FUNCTION FC 90 : VOID
TITLE =GESTIONE ALLARMI / AVVISI
AUTHOR : MassimoZ
VERSION : 0.1

BEGIN
NETWORK
TITLE ======== Avvisi Generali =======



NETWORK
TITLE =Avviso: Manca Marcia Generale
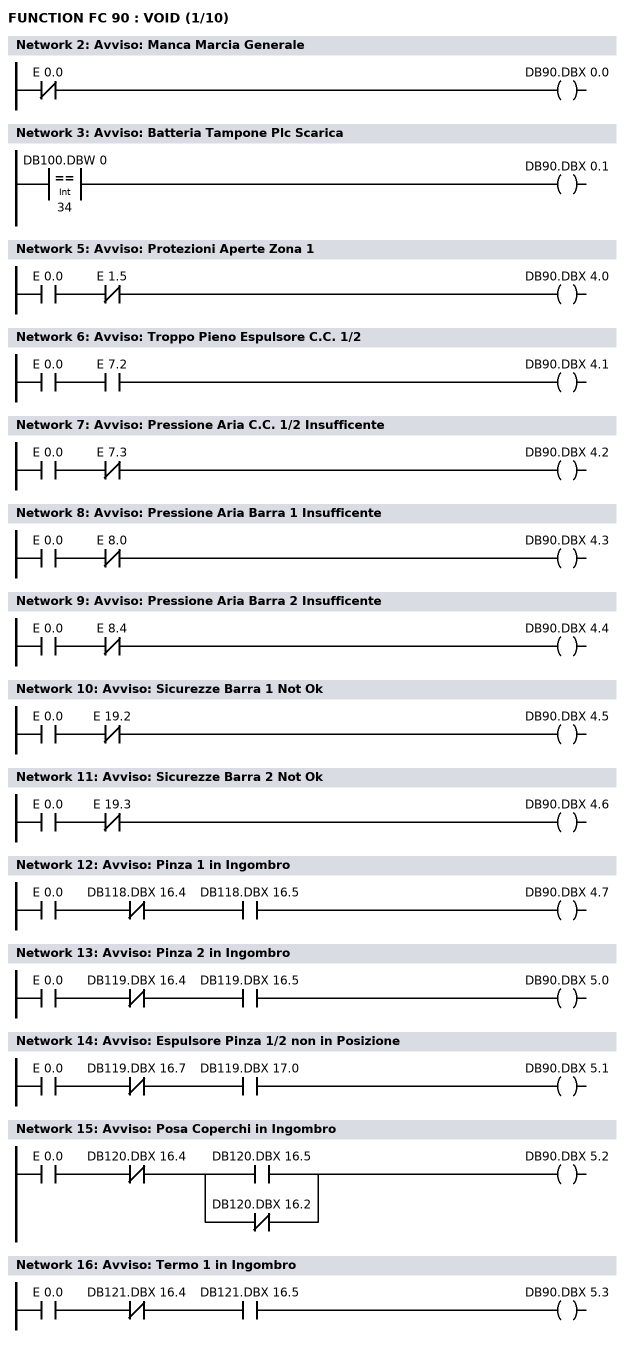
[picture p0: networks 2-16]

      UN    E      0.0;
      =     DB90.DBX    0.0;
NETWORK
TITLE =Avviso: Batteria Tampone Plc Scarica

      L     DB100.DBW    0;
      L     34;
      ==I   ;
      =     DB90.DBX    0.1;
NETWORK
TITLE ======== Avvisi Zona 1 =======



NETWORK
TITLE =Avviso: Protezioni Aperte Zona 1

      U     E      0.0;
      UN    E      1.5;
      =     DB90.DBX    4.0;
NETWORK
TITLE =Avviso: Troppo Pieno Espulsore C.C. 1/2

      U     E      0.0;
      U     E      7.2;
      =     DB90.DBX    4.1;
NETWORK
TITLE =Avviso: Pressione Aria C.C. 1/2 Insufficente

      U     E      0.0;
      UN    E      7.3;
      =     DB90.DBX    4.2;
NETWORK
TITLE =Avviso: Pressione Aria Barra 1 Insufficente

      U     E      0.0;
      UN    E      8.0;
      =     DB90.DBX    4.3;
NETWORK
TITLE =Avviso: Pressione Aria Barra 2 Insufficente

      U     E      0.0;
      UN    E      8.4;
      =     DB90.DBX    4.4;
NETWORK
TITLE =Avviso: Sicurezze Barra 1 Not Ok

      U     E      0.0;
      UN    E     19.2;
      =     DB90.DBX    4.5;
NETWORK
TITLE =Avviso: Sicurezze Barra 2 Not Ok

      U     E      0.0;
      UN    E     19.3;
      =     DB90.DBX    4.6;
NETWORK
TITLE =Avviso: Pinza 1 in Ingombro

      U     E      0.0;
      UN    DB118.DBX   16.4;
      U     DB118.DBX   16.5;
      =     DB90.DBX    4.7;
NETWORK
TITLE =Avviso: Pinza 2 in Ingombro

      U     E      0.0;
      UN    DB119.DBX   16.4;
      U     DB119.DBX   16.5;
      =     DB90.DBX    5.0;
NETWORK
TITLE =Avviso: Espulsore Pinza 1/2 non in Posizione

      U     E      0.0;
      UN    DB119.DBX   16.7;
      U     DB119.DBX   17.0;
      =     DB90.DBX    5.1;
NETWORK
TITLE =Avviso: Posa Coperchi in Ingombro

      U     E      0.0;
      UN    DB120.DBX   16.4;
      U(    ;
      O     DB120.DBX   16.5;
      ON    DB120.DBX   16.2;
      )     ;
      =     DB90.DBX    5.2;
NETWORK
TITLE =Avviso: Termo 1 in Ingombro

      U     E      0.0;
      UN    DB121.DBX   16.4;
      U     DB121.DBX   16.5;
      =     DB90.DBX    5.3;
NETWORK
TITLE =Avviso: Termo 2 in Ingombro
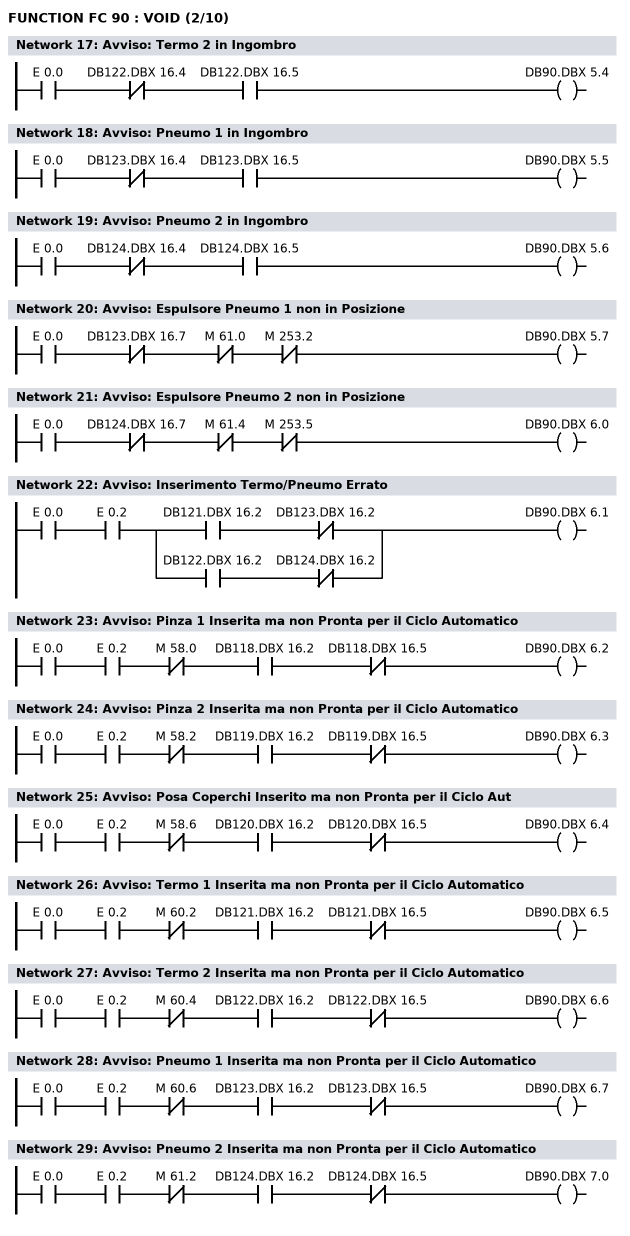
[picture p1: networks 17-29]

      U     E      0.0;
      UN    DB122.DBX   16.4;
      U     DB122.DBX   16.5;
      =     DB90.DBX    5.4;
NETWORK
TITLE =Avviso: Pneumo 1 in Ingombro

      U     E      0.0;
      UN    DB123.DBX   16.4;
      U     DB123.DBX   16.5;
      =     DB90.DBX    5.5;
NETWORK
TITLE =Avviso: Pneumo 2 in Ingombro

      U     E      0.0;
      UN    DB124.DBX   16.4;
      U     DB124.DBX   16.5;
      =     DB90.DBX    5.6;
NETWORK
TITLE =Avviso: Espulsore Pneumo 1 non in Posizione

      U     E      0.0;
      UN    DB123.DBX   16.7;
      UN    M     61.0;
      UN    M    253.2;
      =     DB90.DBX    5.7;
NETWORK
TITLE =Avviso: Espulsore Pneumo 2 non in Posizione

      U     E      0.0;
      UN    DB124.DBX   16.7;
      UN    M     61.4;
      UN    M    253.5;
      =     DB90.DBX    6.0;
NETWORK
TITLE =Avviso: Inserimento Termo/Pneumo Errato

      U     E      0.0;
      U     E      0.2;
      U(    ;
      U     DB121.DBX   16.2;
      UN    DB123.DBX   16.2;
      O     ;
      U     DB122.DBX   16.2;
      UN    DB124.DBX   16.2;
      )     ;
      =     DB90.DBX    6.1;
NETWORK
TITLE =Avviso: Pinza 1 Inserita ma non Pronta per il Ciclo Automatico

      U     E      0.0;
      U     E      0.2;
      UN    M     58.0;
      U     DB118.DBX   16.2;
      UN    DB118.DBX   16.5;
      =     DB90.DBX    6.2;
NETWORK
TITLE =Avviso: Pinza 2 Inserita ma non Pronta per il Ciclo Automatico

      U     E      0.0;
      U     E      0.2;
      UN    M     58.2;
      U     DB119.DBX   16.2;
      UN    DB119.DBX   16.5;
      =     DB90.DBX    6.3;
NETWORK
TITLE =Avviso: Posa Coperchi Inserito ma non Pronta per il Ciclo Aut

      U     E      0.0;
      U     E      0.2;
      UN    M     58.6;
      U     DB120.DBX   16.2;
      UN    DB120.DBX   16.5;
      =     DB90.DBX    6.4;
NETWORK
TITLE =Avviso: Termo 1 Inserita ma non Pronta per il Ciclo Automatico

      U     E      0.0;
      U     E      0.2;
      UN    M     60.2;
      U     DB121.DBX   16.2;
      UN    DB121.DBX   16.5;
      =     DB90.DBX    6.5;
NETWORK
TITLE =Avviso: Termo 2 Inserita ma non Pronta per il Ciclo Automatico

      U     E      0.0;
      U     E      0.2;
      UN    M     60.4;
      U     DB122.DBX   16.2;
      UN    DB122.DBX   16.5;
      =     DB90.DBX    6.6;
NETWORK
TITLE =Avviso: Pneumo 1 Inserita ma non Pronta per il Ciclo Automatico

      U     E      0.0;
      U     E      0.2;
      UN    M     60.6;
      U     DB123.DBX   16.2;
      UN    DB123.DBX   16.5;
      =     DB90.DBX    6.7;
NETWORK
TITLE =Avviso: Pneumo 2 Inserita ma non Pronta per il Ciclo Automatico

      U     E      0.0;
      U     E      0.2;
      UN    M     61.2;
      U     DB124.DBX   16.2;
      UN    DB124.DBX   16.5;
      =     DB90.DBX    7.0;
NETWORK
TITLE =Avviso: Zona Pulsantiera 1 non Pronta per il Ciclo Automatico
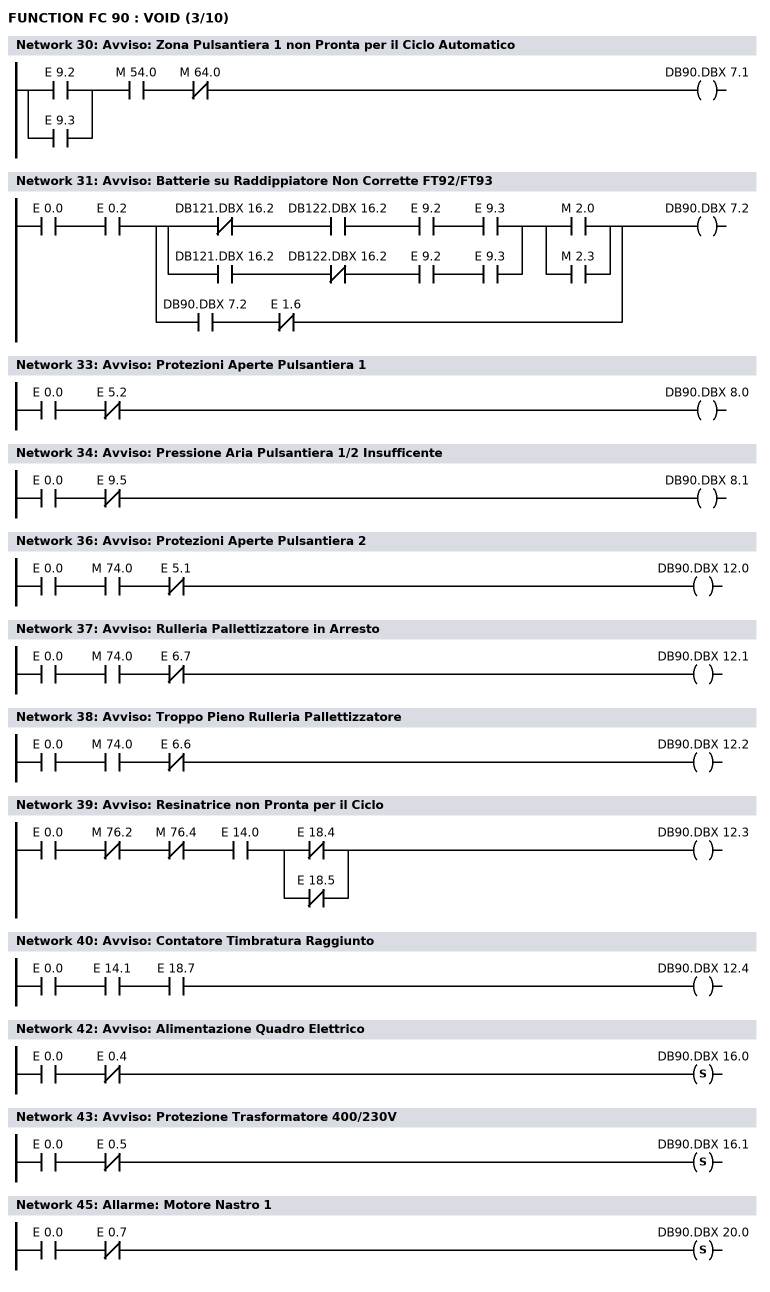
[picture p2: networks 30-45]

      U(    ;
      O     E      9.2;
      O     E      9.3;
      )     ;
      U     M     54.0;
      UN    M     64.0;
      =     DB90.DBX    7.1;
NETWORK
TITLE =Avviso: Batterie su Raddippiatore Non Corrette FT92/FT93

      U     E      0.0;
      U     E      0.2;
      U(    ;
      U(    ;
      UN    DB121.DBX   16.2;
      U     DB122.DBX   16.2;
      U     E      9.2;
      U     E      9.3;
      O     ;
      U     DB121.DBX   16.2;
      UN    DB122.DBX   16.2;
      U     E      9.2;
      U     E      9.3;
      )     ;
      U(    ;
      O     M      2.0;
      O     M      2.3;
      )     ;
      O     ;
      U     DB90.DBX    7.2;
      UN    E      1.6;
      )     ;
      =     DB90.DBX    7.2;
NETWORK
TITLE ======== Avvisi Pulsantiera 1 =======



NETWORK
TITLE =Avviso: Protezioni Aperte Pulsantiera 1

      U     E      0.0;
      UN    E      5.2;
      =     DB90.DBX    8.0;
NETWORK
TITLE =Avviso: Pressione Aria Pulsantiera 1/2 Insufficente

      U     E      0.0;
      UN    E      9.5;
      =     DB90.DBX    8.1;
NETWORK
TITLE ======== Avvisi Pulsantiera 2 =======



NETWORK
TITLE =Avviso: Protezioni Aperte Pulsantiera 2

      U     E      0.0;
      U     M     74.0;
      UN    E      5.1;
      =     DB90.DBX   12.0;
NETWORK
TITLE =Avviso: Rulleria Pallettizzatore in Arresto

      U     E      0.0;
      U     M     74.0;
      UN    E      6.7;
      =     DB90.DBX   12.1;
NETWORK
TITLE =Avviso: Troppo Pieno Rulleria Pallettizzatore

      U     E      0.0;
      U     M     74.0;
      UN    E      6.6;
      =     DB90.DBX   12.2;
NETWORK
TITLE =Avviso: Resinatrice non Pronta per il Ciclo

      U     E      0.0;
      UN    M     76.2;
      UN    M     76.4;
      U     E     14.0;
      U(    ;
      ON    E     18.4;
      ON    E     18.5;
      )     ;
      =     DB90.DBX   12.3;
NETWORK
TITLE =Avviso: Contatore Timbratura Raggiunto

      U     E      0.0;
      U     E     14.1;
      U     E     18.7;
      =     DB90.DBX   12.4;
NETWORK
TITLE ======== Allarmi Generali =======



NETWORK
TITLE =Avviso: Alimentazione Quadro Elettrico

      U     E      0.0;
      UN    E      0.4;
      S     DB90.DBX   16.0;
NETWORK
TITLE =Avviso: Protezione Trasformatore 400/230V

      U     E      0.0;
      UN    E      0.5;
      S     DB90.DBX   16.1;
NETWORK
TITLE ======== Allarmi Zona 1 =======



NETWORK
TITLE =Allarme: Motore Nastro 1

      U     E      0.0;
      UN    E      0.7;
      S     DB90.DBX   20.0;
NETWORK
TITLE =Allarme: Motore Regolazione Altezza C.C.1
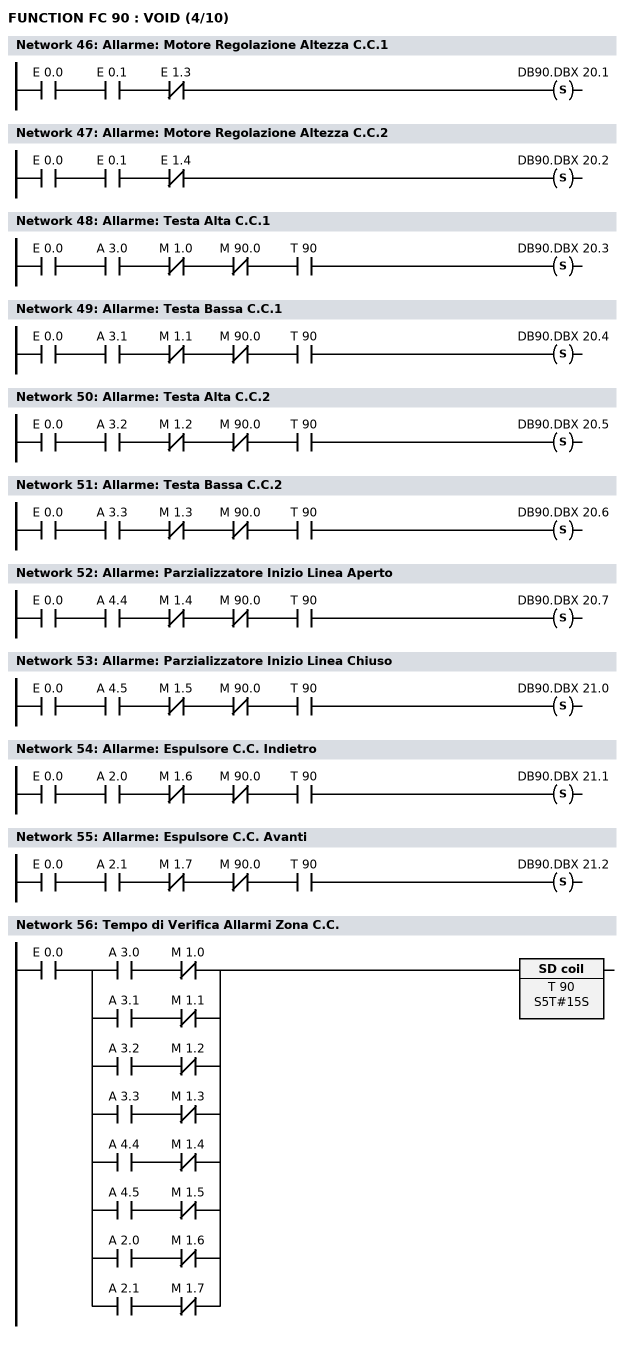
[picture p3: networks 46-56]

      U     E      0.0;
      U     E      0.1;
      UN    E      1.3;
      S     DB90.DBX   20.1;
NETWORK
TITLE =Allarme: Motore Regolazione Altezza C.C.2

      U     E      0.0;
      U     E      0.1;
      UN    E      1.4;
      S     DB90.DBX   20.2;
NETWORK
TITLE =Allarme: Testa Alta C.C.1

      U     E      0.0;
      U     A      3.0;
      UN    M      1.0;
      UN    M     90.0;
      U     T     90;
      S     DB90.DBX   20.3;
NETWORK
TITLE =Allarme: Testa Bassa C.C.1

      U     E      0.0;
      U     A      3.1;
      UN    M      1.1;
      UN    M     90.0;
      U     T     90;
      S     DB90.DBX   20.4;
NETWORK
TITLE =Allarme: Testa Alta C.C.2

      U     E      0.0;
      U     A      3.2;
      UN    M      1.2;
      UN    M     90.0;
      U     T     90;
      S     DB90.DBX   20.5;
NETWORK
TITLE =Allarme: Testa Bassa C.C.2

      U     E      0.0;
      U     A      3.3;
      UN    M      1.3;
      UN    M     90.0;
      U     T     90;
      S     DB90.DBX   20.6;
NETWORK
TITLE =Allarme: Parzializzatore Inizio Linea Aperto

      U     E      0.0;
      U     A      4.4;
      UN    M      1.4;
      UN    M     90.0;
      U     T     90;
      S     DB90.DBX   20.7;
NETWORK
TITLE =Allarme: Parzializzatore Inizio Linea Chiuso

      U     E      0.0;
      U     A      4.5;
      UN    M      1.5;
      UN    M     90.0;
      U     T     90;
      S     DB90.DBX   21.0;
NETWORK
TITLE =Allarme: Espulsore C.C. Indietro

      U     E      0.0;
      U     A      2.0;
      UN    M      1.6;
      UN    M     90.0;
      U     T     90;
      S     DB90.DBX   21.1;
NETWORK
TITLE =Allarme: Espulsore C.C. Avanti

      U     E      0.0;
      U     A      2.1;
      UN    M      1.7;
      UN    M     90.0;
      U     T     90;
      S     DB90.DBX   21.2;
NETWORK
TITLE =Tempo di Verifica Allarmi Zona C.C.

      U     E      0.0;
      U(    ;
      U     A      3.0;
      UN    M      1.0;
      O     ;
      U     A      3.1;
      UN    M      1.1;
      O     ;
      U     A      3.2;
      UN    M      1.2;
      O     ;
      U     A      3.3;
      UN    M      1.3;
      O     ;
      U     A      4.4;
      UN    M      1.4;
      O     ;
      U     A      4.5;
      UN    M      1.5;
      O     ;
      U     A      2.0;
      UN    M      1.6;
      O     ;
      U     A      2.1;
      UN    M      1.7;
      )     ;
      L     S5T#15S;
      SE    T     90;
NETWORK
TITLE =Presenza Allarme Barra 1/2
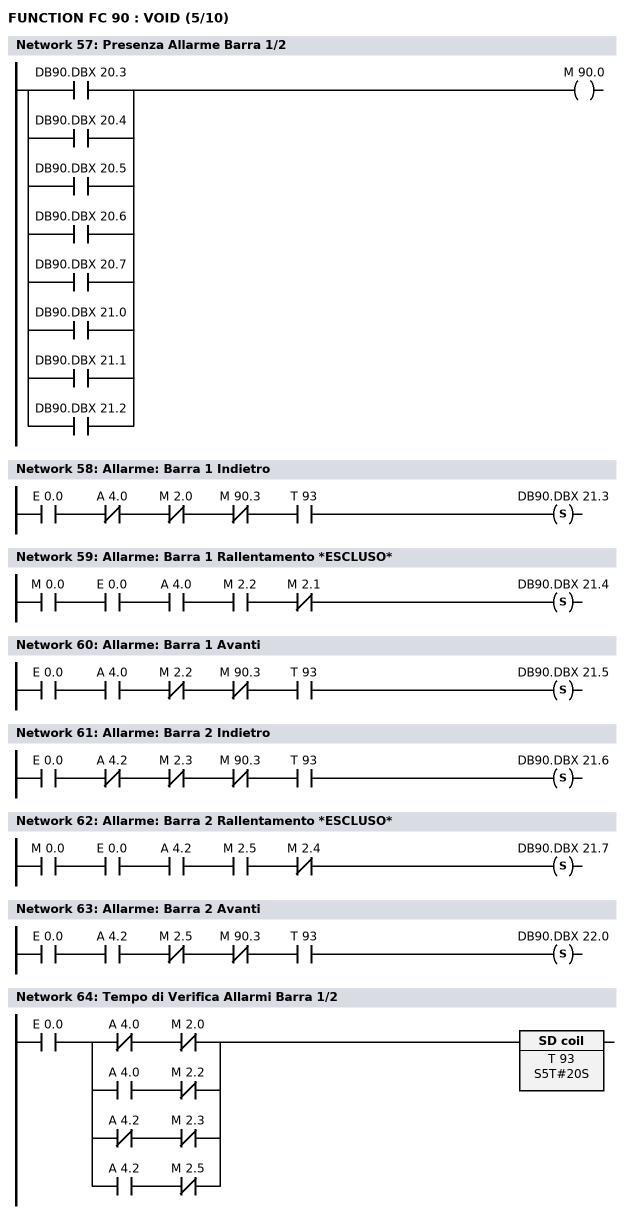
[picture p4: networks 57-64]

      O     DB90.DBX   20.3;
      O     DB90.DBX   20.4;
      O     DB90.DBX   20.5;
      O     DB90.DBX   20.6;
      O     DB90.DBX   20.7;
      O     DB90.DBX   21.0;
      O     DB90.DBX   21.1;
      O     DB90.DBX   21.2;
      =     M     90.0;
NETWORK
TITLE =Allarme: Barra 1 Indietro

      U     E      0.0;
      UN    A      4.0;
      UN    M      2.0;
      UN    M     90.3;
      U     T     93;
      S     DB90.DBX   21.3;
NETWORK
TITLE =Allarme: Barra 1 Rallentamento *ESCLUSO*

      U     M      0.0;
      U     E      0.0;
      U     A      4.0;
      U     M      2.2;
      UN    M      2.1;
      S     DB90.DBX   21.4;
NETWORK
TITLE =Allarme: Barra 1 Avanti

      U     E      0.0;
      U     A      4.0;
      UN    M      2.2;
      UN    M     90.3;
      U     T     93;
      S     DB90.DBX   21.5;
NETWORK
TITLE =Allarme: Barra 2 Indietro

      U     E      0.0;
      UN    A      4.2;
      UN    M      2.3;
      UN    M     90.3;
      U     T     93;
      S     DB90.DBX   21.6;
NETWORK
TITLE =Allarme: Barra 2 Rallentamento *ESCLUSO*

      U     M      0.0;
      U     E      0.0;
      U     A      4.2;
      U     M      2.5;
      UN    M      2.4;
      S     DB90.DBX   21.7;
NETWORK
TITLE =Allarme: Barra 2 Avanti

      U     E      0.0;
      U     A      4.2;
      UN    M      2.5;
      UN    M     90.3;
      U     T     93;
      S     DB90.DBX   22.0;
NETWORK
TITLE =Tempo di Verifica Allarmi Barra 1/2

      U     E      0.0;
      U(    ;
      UN    A      4.0;
      UN    M      2.0;
      O     ;
      U     A      4.0;
      UN    M      2.2;
      O     ;
      UN    A      4.2;
      UN    M      2.3;
      O     ;
      U     A      4.2;
      UN    M      2.5;
      )     ;
      L     S5T#20S;
      SE    T     93;
NETWORK
TITLE =Presenza Allarme Barra 1/2
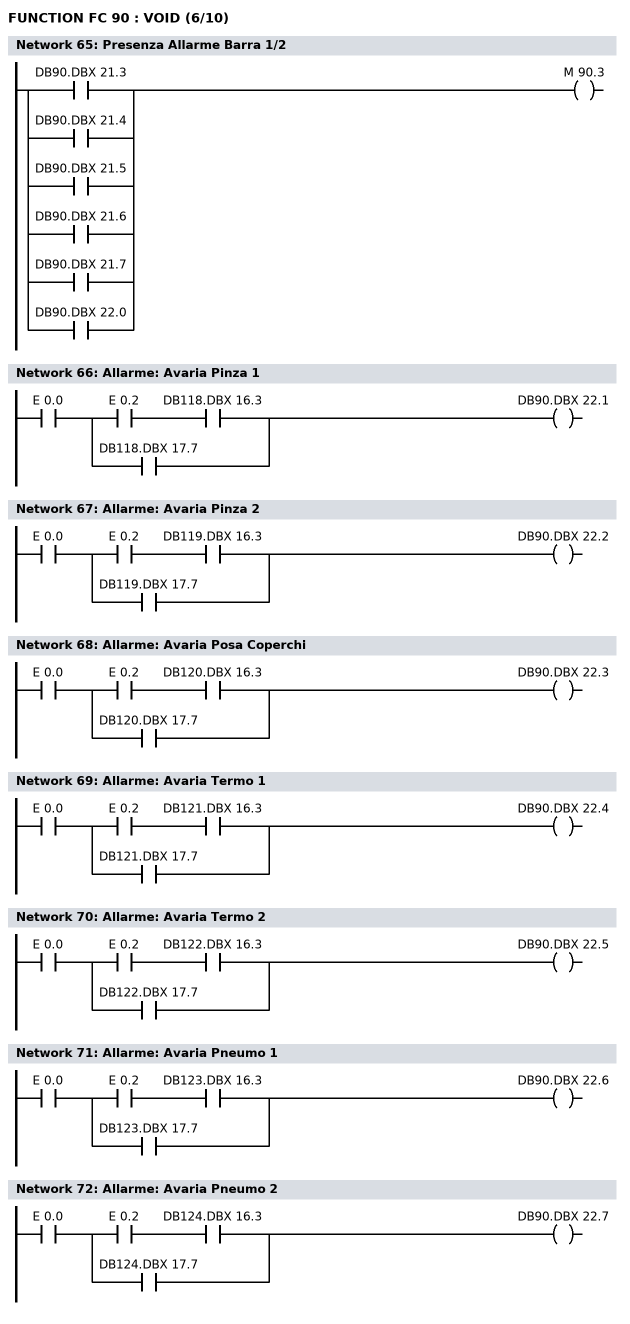
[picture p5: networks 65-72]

      O     DB90.DBX   21.3;
      O     DB90.DBX   21.4;
      O     DB90.DBX   21.5;
      O     DB90.DBX   21.6;
      O     DB90.DBX   21.7;
      O     DB90.DBX   22.0;
      =     M     90.3;
NETWORK
TITLE =Allarme: Avaria Pinza 1

      U     E      0.0;
      U(    ;
      U     E      0.2;
      U     DB118.DBX   16.3;
      O     DB118.DBX   17.7;
      )     ;
      =     DB90.DBX   22.1;
NETWORK
TITLE =Allarme: Avaria Pinza 2

      U     E      0.0;
      U(    ;
      U     E      0.2;
      U     DB119.DBX   16.3;
      O     DB119.DBX   17.7;
      )     ;
      =     DB90.DBX   22.2;
NETWORK
TITLE =Allarme: Avaria Posa Coperchi

      U     E      0.0;
      U(    ;
      U     E      0.2;
      U     DB120.DBX   16.3;
      O     DB120.DBX   17.7;
      )     ;
      =     DB90.DBX   22.3;
NETWORK
TITLE =Allarme: Avaria Termo 1

      U     E      0.0;
      U(    ;
      U     E      0.2;
      U     DB121.DBX   16.3;
      O     DB121.DBX   17.7;
      )     ;
      =     DB90.DBX   22.4;
NETWORK
TITLE =Allarme: Avaria Termo 2

      U     E      0.0;
      U(    ;
      U     E      0.2;
      U     DB122.DBX   16.3;
      O     DB122.DBX   17.7;
      )     ;
      =     DB90.DBX   22.5;
NETWORK
TITLE =Allarme: Avaria Pneumo 1

      U     E      0.0;
      U(    ;
      U     E      0.2;
      U     DB123.DBX   16.3;
      O     DB123.DBX   17.7;
      )     ;
      =     DB90.DBX   22.6;
NETWORK
TITLE =Allarme: Avaria Pneumo 2

      U     E      0.0;
      U(    ;
      U     E      0.2;
      U     DB124.DBX   16.3;
      O     DB124.DBX   17.7;
      )     ;
      =     DB90.DBX   22.7;
NETWORK
TITLE ======== Allarmi Pulsantiera 1 =======



NETWORK
TITLE =Allarme: Inverter
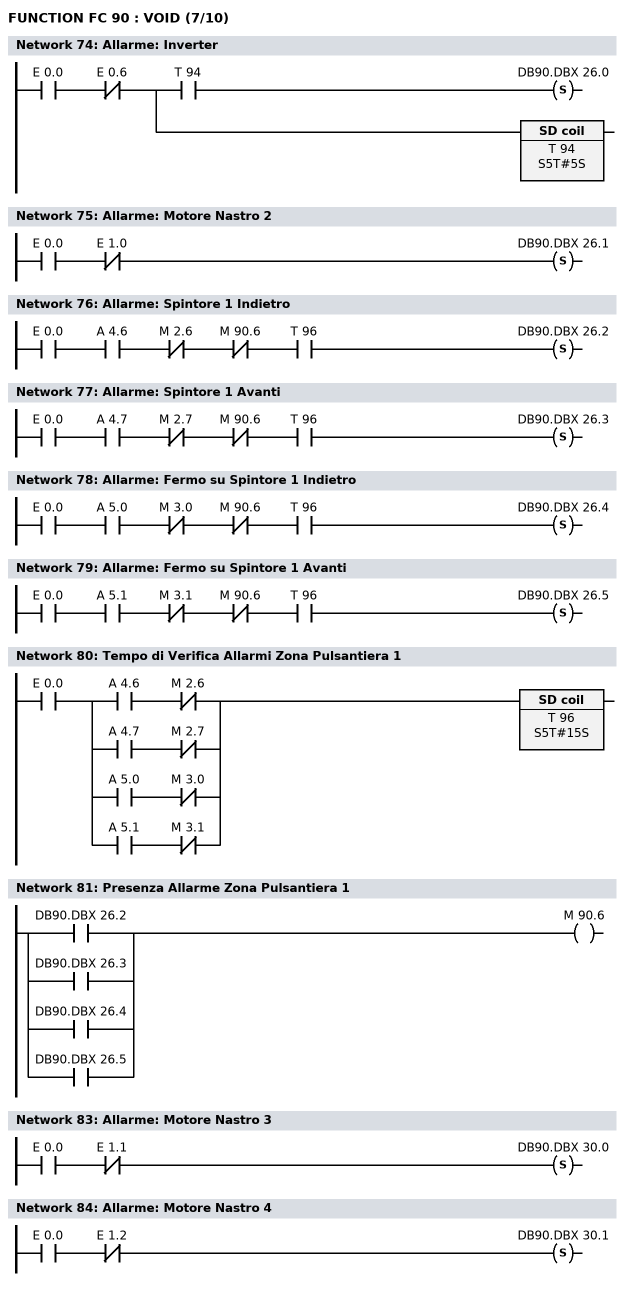
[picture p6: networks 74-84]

      U     E      0.0;
      UN    E      0.6;
      =     L      0.0;
      U     L      0.0;
      U     T     94;
      S     DB90.DBX   26.0;
      U     L      0.0;
      BLD   102;
      L     S5T#5S;
      SE    T     94;
NETWORK
TITLE =Allarme: Motore Nastro 2

      U     E      0.0;
      UN    E      1.0;
      S     DB90.DBX   26.1;
NETWORK
TITLE =Allarme: Spintore 1 Indietro

      U     E      0.0;
      U     A      4.6;
      UN    M      2.6;
      UN    M     90.6;
      U     T     96;
      S     DB90.DBX   26.2;
NETWORK
TITLE =Allarme: Spintore 1 Avanti

      U     E      0.0;
      U     A      4.7;
      UN    M      2.7;
      UN    M     90.6;
      U     T     96;
      S     DB90.DBX   26.3;
NETWORK
TITLE =Allarme: Fermo su Spintore 1 Indietro

      U     E      0.0;
      U     A      5.0;
      UN    M      3.0;
      UN    M     90.6;
      U     T     96;
      S     DB90.DBX   26.4;
NETWORK
TITLE =Allarme: Fermo su Spintore 1 Avanti

      U     E      0.0;
      U     A      5.1;
      UN    M      3.1;
      UN    M     90.6;
      U     T     96;
      S     DB90.DBX   26.5;
NETWORK
TITLE =Tempo di Verifica Allarmi Zona Pulsantiera 1

      U     E      0.0;
      U(    ;
      U     A      4.6;
      UN    M      2.6;
      O     ;
      U     A      4.7;
      UN    M      2.7;
      O     ;
      U     A      5.0;
      UN    M      3.0;
      O     ;
      U     A      5.1;
      UN    M      3.1;
      )     ;
      L     S5T#15S;
      SE    T     96;
NETWORK
TITLE =Presenza Allarme Zona Pulsantiera 1

      O     DB90.DBX   26.2;
      O     DB90.DBX   26.3;
      O     DB90.DBX   26.4;
      O     DB90.DBX   26.5;
      =     M     90.6;
NETWORK
TITLE ======== Allarmi Pulsantiera 2 =======



NETWORK
TITLE =Allarme: Motore Nastro 3

      U     E      0.0;
      UN    E      1.1;
      S     DB90.DBX   30.0;
NETWORK
TITLE =Allarme: Motore Nastro 4

      U     E      0.0;
      UN    E      1.2;
      S     DB90.DBX   30.1;
NETWORK
TITLE =Allarme: Parzializzatore SX Nastro 3 Aperto
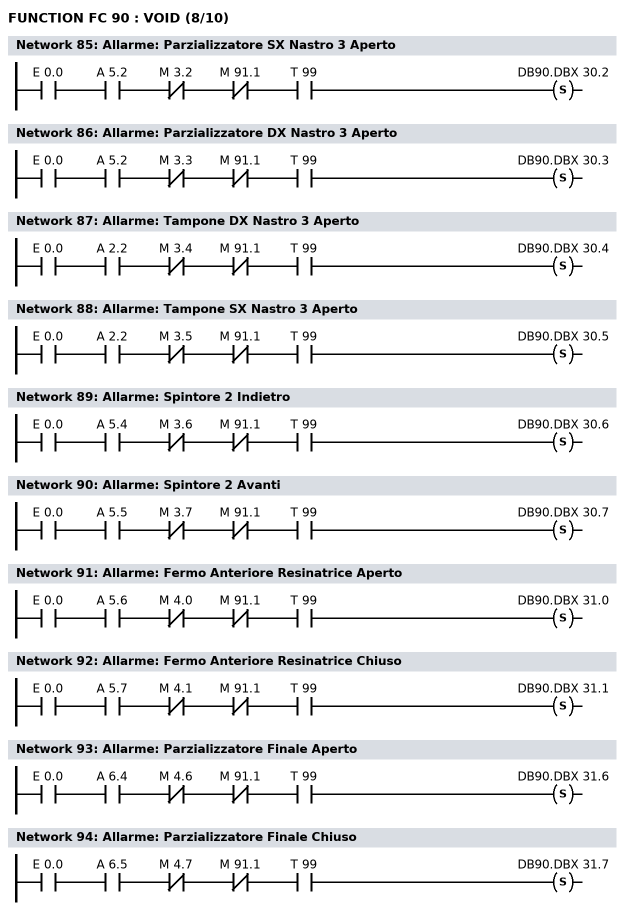
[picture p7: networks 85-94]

      U     E      0.0;
      U     A      5.2;
      UN    M      3.2;
      UN    M     91.1;
      U     T     99;
      S     DB90.DBX   30.2;
NETWORK
TITLE =Allarme: Parzializzatore DX Nastro 3 Aperto

      U     E      0.0;
      U     A      5.2;
      UN    M      3.3;
      UN    M     91.1;
      U     T     99;
      S     DB90.DBX   30.3;
NETWORK
TITLE =Allarme: Tampone DX Nastro 3 Aperto

      U     E      0.0;
      U     A      2.2;
      UN    M      3.4;
      UN    M     91.1;
      U     T     99;
      S     DB90.DBX   30.4;
NETWORK
TITLE =Allarme: Tampone SX Nastro 3 Aperto

      U     E      0.0;
      U     A      2.2;
      UN    M      3.5;
      UN    M     91.1;
      U     T     99;
      S     DB90.DBX   30.5;
NETWORK
TITLE =Allarme: Spintore 2 Indietro

      U     E      0.0;
      U     A      5.4;
      UN    M      3.6;
      UN    M     91.1;
      U     T     99;
      S     DB90.DBX   30.6;
NETWORK
TITLE =Allarme: Spintore 2 Avanti

      U     E      0.0;
      U     A      5.5;
      UN    M      3.7;
      UN    M     91.1;
      U     T     99;
      S     DB90.DBX   30.7;
NETWORK
TITLE =Allarme: Fermo Anteriore Resinatrice Aperto

      U     E      0.0;
      U     A      5.6;
      UN    M      4.0;
      UN    M     91.1;
      U     T     99;
      S     DB90.DBX   31.0;
NETWORK
TITLE =Allarme: Fermo Anteriore Resinatrice Chiuso

      U     E      0.0;
      U     A      5.7;
      UN    M      4.1;
      UN    M     91.1;
      U     T     99;
      S     DB90.DBX   31.1;
NETWORK
TITLE =Allarme: Parzializzatore Finale Aperto

      U     E      0.0;
      U     A      6.4;
      UN    M      4.6;
      UN    M     91.1;
      U     T     99;
      S     DB90.DBX   31.6;
NETWORK
TITLE =Allarme: Parzializzatore Finale Chiuso

      U     E      0.0;
      U     A      6.5;
      UN    M      4.7;
      UN    M     91.1;
      U     T     99;
      S     DB90.DBX   31.7;
NETWORK
TITLE =Tempo di Verifica Allarmi Parz/Fermi Zona Pulsantiera 2
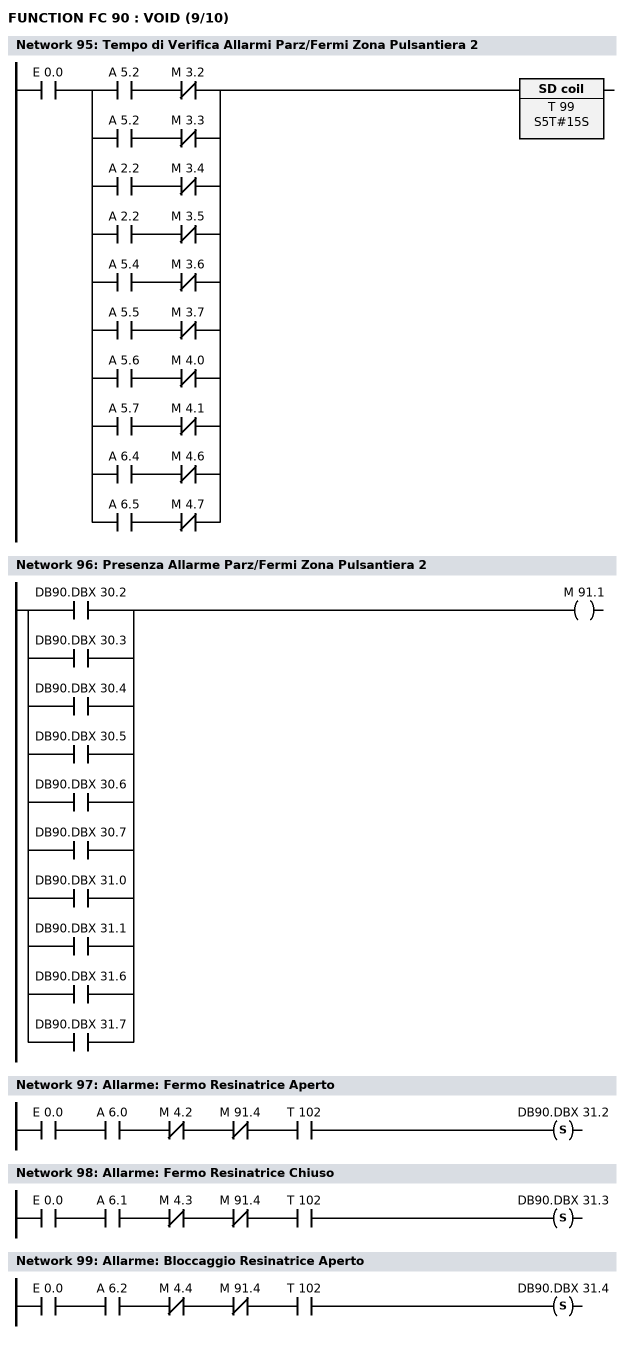
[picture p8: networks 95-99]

      U     E      0.0;
      U(    ;
      U     A      5.2;
      UN    M      3.2;
      O     ;
      U     A      5.2;
      UN    M      3.3;
      O     ;
      U     A      2.2;
      UN    M      3.4;
      O     ;
      U     A      2.2;
      UN    M      3.5;
      O     ;
      U     A      5.4;
      UN    M      3.6;
      O     ;
      U     A      5.5;
      UN    M      3.7;
      O     ;
      U     A      5.6;
      UN    M      4.0;
      O     ;
      U     A      5.7;
      UN    M      4.1;
      O     ;
      U     A      6.4;
      UN    M      4.6;
      O     ;
      U     A      6.5;
      UN    M      4.7;
      )     ;
      L     S5T#15S;
      SE    T     99;
NETWORK
TITLE =Presenza Allarme Parz/Fermi Zona Pulsantiera 2

      O     DB90.DBX   30.2;
      O     DB90.DBX   30.3;
      O     DB90.DBX   30.4;
      O     DB90.DBX   30.5;
      O     DB90.DBX   30.6;
      O     DB90.DBX   30.7;
      O     DB90.DBX   31.0;
      O     DB90.DBX   31.1;
      O     DB90.DBX   31.6;
      O     DB90.DBX   31.7;
      =     M     91.1;
NETWORK
TITLE =Allarme: Fermo Resinatrice Aperto

      U     E      0.0;
      U     A      6.0;
      UN    M      4.2;
      UN    M     91.4;
      U     T    102;
      S     DB90.DBX   31.2;
NETWORK
TITLE =Allarme: Fermo Resinatrice Chiuso

      U     E      0.0;
      U     A      6.1;
      UN    M      4.3;
      UN    M     91.4;
      U     T    102;
      S     DB90.DBX   31.3;
NETWORK
TITLE =Allarme: Bloccaggio Resinatrice Aperto

      U     E      0.0;
      U     A      6.2;
      UN    M      4.4;
      UN    M     91.4;
      U     T    102;
      S     DB90.DBX   31.4;
NETWORK
TITLE =Allarme: Bloccaggio Resinatrice Chiuso
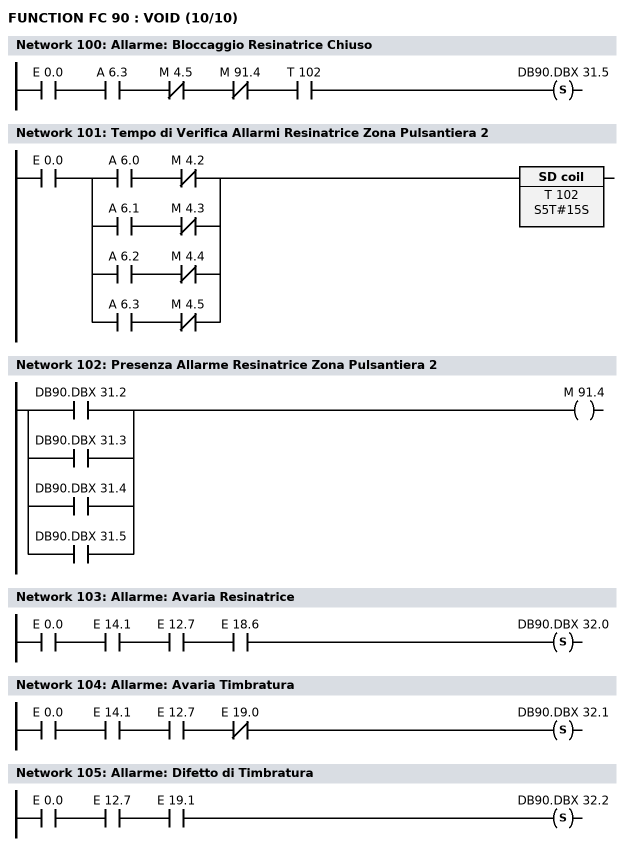
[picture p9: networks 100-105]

      U     E      0.0;
      U     A      6.3;
      UN    M      4.5;
      UN    M     91.4;
      U     T    102;
      S     DB90.DBX   31.5;
NETWORK
TITLE =Tempo di Verifica Allarmi Resinatrice Zona Pulsantiera 2

      U     E      0.0;
      U(    ;
      U     A      6.0;
      UN    M      4.2;
      O     ;
      U     A      6.1;
      UN    M      4.3;
      O     ;
      U     A      6.2;
      UN    M      4.4;
      O     ;
      U     A      6.3;
      UN    M      4.5;
      )     ;
      L     S5T#15S;
      SE    T    102;
NETWORK
TITLE =Presenza Allarme Resinatrice Zona Pulsantiera 2

      O     DB90.DBX   31.2;
      O     DB90.DBX   31.3;
      O     DB90.DBX   31.4;
      O     DB90.DBX   31.5;
      =     M     91.4;
NETWORK
TITLE =Allarme: Avaria Resinatrice

      U     E      0.0;
      U     E     14.1;
      U     E     12.7;
      U     E     18.6;
      S     DB90.DBX   32.0;
NETWORK
TITLE =Allarme: Avaria Timbratura

      U     E      0.0;
      U     E     14.1;
      U     E     12.7;
      UN    E     19.0;
      S     DB90.DBX   32.1;
NETWORK
TITLE =Allarme: Difetto di Timbratura

      U     E      0.0;
      U     E     12.7;
      U     E     19.1;
      S     DB90.DBX   32.2;
NETWORK
TITLE =Reset Allarmi Generali e 1a Zona

      U     E      1.6;
      FP    DB100.DBX   12.0;
      SPBNB RA1;
      L     0;
      T     DB90.DBW   16;
      T     DB90.DBW   18;
      T     DB90.DBW   20;
      T     DB90.DBW   22;
      T     DB90.DBW   24;
RA1:  NOP   0;

//ACQUISIZIONE ALLARMI DA PLC
//----------
      L     DB90.DBW   16;
      INVI  ;
      T     DB90.DBW   36;
//----------
      L     DB90.DBW   18;
      INVI  ;
      T     DB90.DBW   38;
//----------
      L     DB90.DBW   20;
      INVI  ;
      T     DB90.DBW   40;
//----------
      L     DB90.DBW   22;
      INVI  ;
      T     DB90.DBW   42;
//----------
      L     DB90.DBW   24;
      INVI  ;
      T     DB90.DBW   44;
//----------
NETWORK
TITLE =Reset Allarmi Pulsantiera 1

      U     E     10.4;
      FP    DB100.DBX   12.1;
      SPBNB RA2;
      L     0;
      T     DB90.DBW   26;
      T     DB90.DBW   28;
RA2:  NOP   0;

//ACQUISIZIONE ALLARMI DA PLC
//----------
      L     DB90.DBW   26;
      INVI  ;
      T     DB90.DBW   46;
//----------
      L     DB90.DBW   28;
      INVI  ;
      T     DB90.DBW   48;
//----------
NETWORK
TITLE =Reset Allarmi Pulsantiera 2

      U     E     13.4;
      FP    DB100.DBX   12.2;
      SPBNB RA3;
      L     0;
      T     DB90.DBW   30;
      T     DB90.DBW   32;
      T     DB90.DBW   34;
RA3:  NOP   0;

//ACQUISIZIONE ALLARMI DA PLC
//----------
      L     DB90.DBW   30;
      INVI  ;
      T     DB90.DBW   50;
//----------
      L     DB90.DBW   32;
      INVI  ;
      T     DB90.DBW   52;
//----------
      L     DB90.DBW   34;
      INVI  ;
      T     DB90.DBW   54;
//----------
END_FUNCTION

